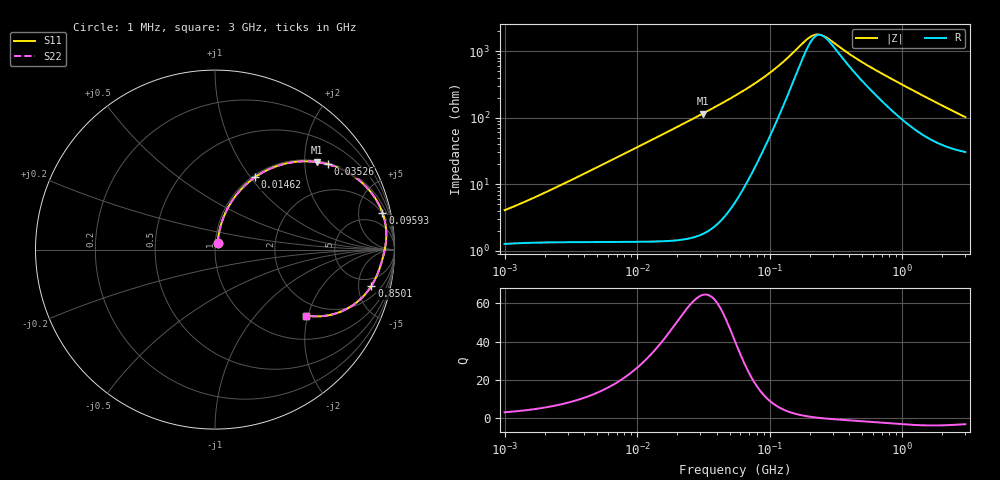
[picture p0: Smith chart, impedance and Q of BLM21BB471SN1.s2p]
! BLM21BB471SN1
# Hz S RI R 50
!Freq.(Hz) S11(Real) S11(Imag) S21(Real) S21(Imag) S12(Real) S12(Imag) S22(Real) S22(Imag)
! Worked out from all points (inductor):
!   401 points, 1 MHz to 3 GHz, reference 50 ohm
!   read as one part in series: L = 597 nH near 1.041 MHz
!   highest Q = 64.4 at 31.27 MHz (marker M1), where L = 585 nH
!   self-resonance near 244.8 MHz
!   S11 on the Smith chart (normalised r, x): 1 MHz: 1.03, +0.08; 14.62 MHz: 1.03, +1.05; 35.26 MHz: 1.04, +2.61; 95.93 MHz: 1.86, +8.77; 850.1 MHz: 3.48, -7.03; 3 GHz: 1.61, -1.94
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1000000  0.014 0.0376  0.986 -0.0376  0.986 -0.0376  0.014 0.0376
2097170  0.0187 0.074  0.9813 -0.074  0.9813 -0.074  0.0187 0.074
3823119  0.0311 0.1314  0.9689 -0.1314  0.9689 -0.1314  0.0311 0.1314
8179831  0.0895 0.2633  0.9105 -0.2633  0.9105 -0.2633  0.0895 0.2633
1.461624e7  0.2225 0.403  0.7775 -0.403  0.7775 -0.403  0.2225 0.403
2.225279e7  0.396 0.48  0.604 -0.48  0.604 -0.48  0.396 0.48
3.127247e7  0.568 0.4876  0.432 -0.4876  0.432 -0.4876  0.568 0.4876
3.526298e7  0.6283 0.4755  0.3717 -0.4755  0.3717 -0.4755  0.6283 0.4755
5.477226e7  0.8135 0.3772  0.1865 -0.3772  0.1865 -0.3772  0.8135 0.3772
7.248696e7  0.8891 0.2916  0.1109 -0.2916  0.1109 -0.2916  0.8891 0.2916
9.593103e7  0.9327 0.2061  0.0673 -0.2061  0.0673 -0.2061  0.9327 0.2061
1.244416e8  0.9508 0.1351  0.0492 -0.1351  0.0492 -0.1351  0.9508 0.1351
1.857042e8  0.9528 0.0474  0.0472 -0.0474  0.0472 -0.0474  0.9528 0.0474
2.094008e8  0.9502 0.0257  0.0498 -0.0257  0.0498 -0.0257  0.9502 0.0257
2.314421e8  0.9474 0.00898  0.0526 -0.00898  0.0526 -0.00898  0.9474 0.00898
2.609752e8  0.9436 -0.00998  0.0564 0.00998  0.0564 0.00998  0.9436 -0.00998
4.570858e8  0.921 -0.0929  0.079 0.0929  0.079 0.0929  0.921 -0.0929
8.005644e8  0.8784 -0.1903  0.1216 0.1903  0.1216 0.1903  0.8784 -0.1903
8.501091e8  0.8712 -0.2023  0.1288 0.2023  0.1288 0.2023  0.8712 -0.2023
1.488926e9  0.7577 -0.3166  0.2423 0.3166  0.2423 0.3166  0.7577 -0.3166
2.134733e9  0.6365 -0.3651  0.3635 0.3651  0.3635 0.3651  0.6365 -0.3651
3e9  0.5068 -0.3673  0.4932 0.3673  0.4932 0.3673  0.5068 -0.3673
